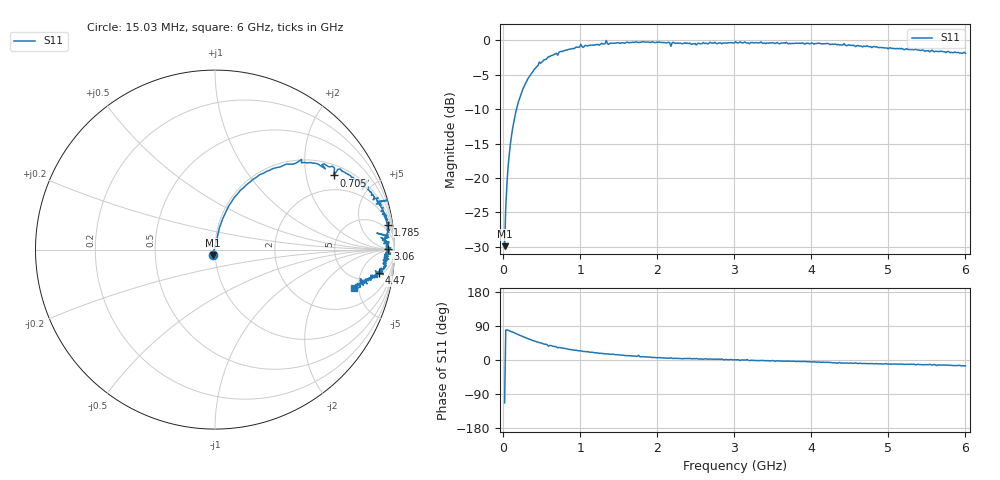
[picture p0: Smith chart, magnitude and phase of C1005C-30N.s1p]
!	Network	Analyzer	HP8753E.07.74:	Oct	30	2002	Serial	No.	JP38451487
!	Hewlett-Packard
!	7	Sep	2009	9:02:54
!	Frequency	S11
#	HZ	S	RI	R	50
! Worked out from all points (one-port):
!   400 points, 15.03 MHz to 6 GHz, reference 50 ohm
!   lowest |S11| = -29.9 dB at 15.03 MHz (marker M1), VSWR 1.07, Z = 48.7 - j2.86 ohm
!   |S11| at or under -10 dB: start of sweep to 169.8 MHz
!   S11 on the Smith chart (normalised r, x): 15.03 MHz: 0.97, -0.06; 705 MHz: 1.37, +2.90; 1.785 GHz: 3, +13; 3.06 GHz: 54, +5; 4.47 GHz: 6, -11; 6 GHz: 3.65, -4.48
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1.502992e7  -0.0126 -0.0293
3.002985e7  0.0115 0.0603
7.502962e7  0.0328 0.144
1.200294e8  0.0656 0.221
1.95029e8  0.141 0.33
4.650277e8  0.482 0.502
5.850271e8  0.615 0.45
7.050265e8  0.662 0.413
7.650262e8  0.705 0.438
1.005025e9  0.854 0.385
1.320023e9  0.907 0.269
1.335023e9  0.961 0.275
1.365023e9  0.899 0.254
1.515022e9  0.925 0.214
1.740021e9  0.958 0.163
1.755021e9  0.942 0.208
1.785021e9  0.962 0.139
2.145019e9  0.965 0.0813
2.175019e9  0.902 0.0919
2.205019e9  0.968 0.0673
2.265019e9  0.956 0.0704
3.015015e9  0.979 0.0103
3.060015e9  0.964 0.00314
3.765011e9  0.948 -0.0505
4.470008e9  0.912 -0.131
4.515007e9  0.913 -0.13
5.265004e9  0.844 -0.171
6e9  0.777 -0.215
